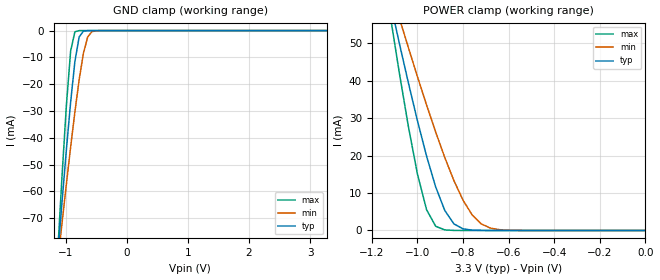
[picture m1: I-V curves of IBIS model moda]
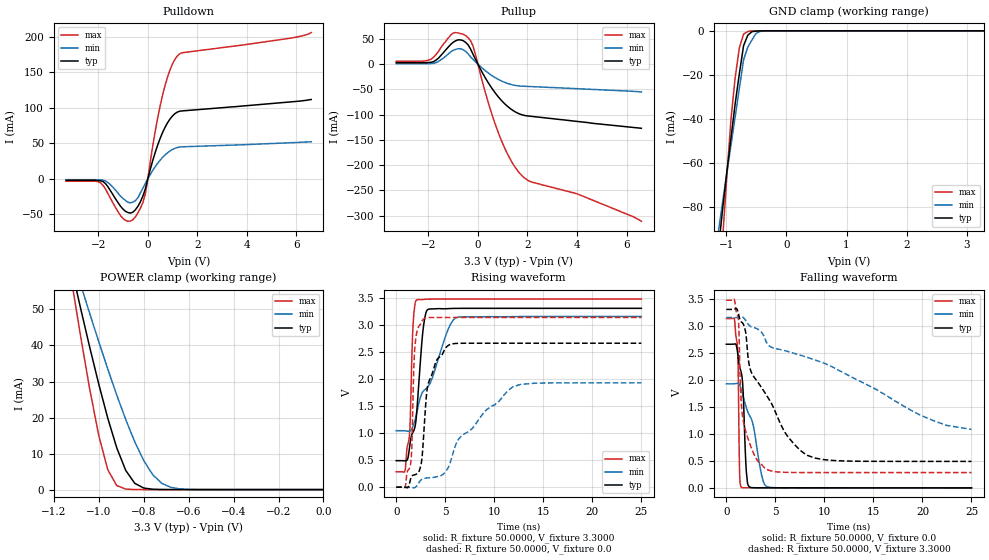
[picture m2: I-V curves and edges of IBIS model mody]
| IBIS (I/O, Buffer, Information, Specification) Model, officially
| electronic behavioral standard for Buffer structures of digital pins.
[IBIS ver]  4.0
[File name] 54ac04_3v3_rev1.ibs
[File Rev]  1.0
[Date]   4 Oct 2017
[Source]   CAD & Design Services (Catania) - STMicroelectronics
[Notes]
  (Note1) This IBIS model is the model of the product with package
   (Flat14 package elements);
  (Note2) This IBIS model is extracted with nominal 3.3V power supply
   (min:3.15V, typ:3.3V, max:3.47V);
  (Note3) This model has few Warnings about the non-monotonicity
   of I-V curves, but they are not indicative of problems
   inside the model;
[Copyright] (c) 2017 STMicroelectronics
|   Component 54AC04
[Component] 54AC04
[Manufacturer] STMicroelectronics
[Package]
| variable   typ   min   max
R_pkg   0.0   0.0   0.0
L_pkg   0.0H   0.0H   0.0H
C_pkg   0.0F   0.0F   0.0F
[Pin]  signal_name   model_name   R_pin   L_pin   C_pin
1   A0   moda   141.0m   4.31nH   1.01pF
2   O0   mody   108.1m   3.05nH   1.04pF
3   A1   moda   90.5m   2.36nH   0.8pF
4   O1   mody   79.7m   1.96nH   0.8pF
5   A2   moda   86.2m   2.16nH   0.8pF
6   O2   mody   101.7m   2.85nH   1.04pF
7   GND   GND   111.0m   3.51nH   1.01pF
8   O5   mody   141.0m   4.31nH   1.01pF
9   A5   moda   112.4m   3.25nH   1.04pF
10   O4   mody   90.5m   2.36nH   0.8pF
11   A4   moda   81.9m   2.06nH   0.8pF
12   O3   mody   84.0m   2.16nH   0.8pF
13   A3   moda   101.7m   2.85nH   1.04pF
14   VCC   POWER   111.0m   3.51nH   1.01pF
| Models and submodels in the file (2): moda (Input), mody (I/O)
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|   Model mod_a
[Model]   moda
Model_type Input
Vinl   =   1.000V
Vinh   =   2.300V
C_comp   0.584pF   0.443pF   0.735pF
[Temperature Range]  25.0000   0.1250k   -55.0000
[Voltage Range]   3.3000V   3.1500V   3.4700V
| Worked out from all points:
|   GND clamp passes 1 mA (typ) near -0.74 V on its own axis
|   POWER clamp passes 1 mA (typ) near -0.82 V on its own axis
[GND_clamp]
|Voltage   I(typ)   I(min)   I(max)
-3.3V     -749mA     -568.4mA   -1.036A
-1.13V    -83.59mA   -86.25mA   -82mA
-1.06V    -63.75mA   -71.67mA   -54.05mA
-990mV    -44.61mA   -57.39mA   -28.12mA
-920mV    -26.72mA   -43.53mA   -7.666mA
-850mV    -11.52mA   -30.35mA   -438.9uA
-780mV    -2.357mA   -18.3mA    -11.16uA
-710mV    -202.6uA   -8.405mA   -269.9nA
-640mV    -13.61uA   -2.367mA   -6.525nA
-570mV    -893.7nA   -396.6uA   -166.8pA
-430mV    -3.851nA   -7.049uA   -9.012pA
3.28V     6.52pA     5.985nA    5.92pA
[POWER_clamp]
|Voltage   I(typ)   I(min)   I(max)
-3.28V    721.1mA    542.9mA    1.005A
-1.12V    61.08mA    64.91mA    57.6mA
-1.08V    50.1mA     56.8mA     42.24mA
-1.04V    39.44mA    48.83mA    27.8mA
-1V       29.27mA    41.04mA    15.03mA
-960mV    19.83mA    33.48mA    5.531mA
-920mV    11.6mA     26.24mA    1.117mA
-880mV    5.324mA    19.45mA    149.5uA
-840mV    1.752mA    13.29mA    18.09uA
-760mV    95.86uA    4.148mA    257.2nA
-680mV    4.309uA    633uA      3.657nA
0V        6.6pA      45.39pA    7.2pA
|   Model mody
[Model]   mody
Model_type I/O
Polarity   Inverting
Vinl   =   1.000V
Vinh   =   2.300V
Vmeas  =   1.650V
Cref   =   50pf
Rref   =   500
C_comp   3.516pF   2.793pF   4.427pF
[Temperature Range]  25.0000   0.1250k   -55.0000
[Voltage Range]   3.3000V   3.1500V   3.4700V
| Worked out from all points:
|   slope of the pulldown table from 0 to 0.495 V, typ, clamps not added: 8.73 ohm
|   slope of the pullup table from 0 to 0.495 V, typ, clamps not added: 11.6 ohm
|   GND clamp passes 1 mA (typ) near -0.60 V on its own axis
|   POWER clamp passes 1 mA (typ) near -0.82 V on its own axis
|   rising waveform, R_fixture 50.0000, V_fixture 3.3000: 20-80 % time 832ps typ, 2.72ns min, 347ps max; typ from 0.489 V to 3.3 V
|   rising waveform, R_fixture 50.0000, V_fixture 0.0: 20-80 % time 1.1ns typ, 4.82ns min, 312ps max; typ from 0 V to 2.66 V
|   falling waveform, R_fixture 50.0000, V_fixture 0.0: 20-80 % time 438ps typ, 1.49ns min, 152ps max; typ from 2.66 V to 0 V
|   falling waveform, R_fixture 50.0000, V_fixture 3.3000: 20-80 % time 3.84ns typ, 14.3ns min, 894ps max; typ from 3.3 V to 0.489 V
[Pulldown]
|Voltage   I(typ)   I(min)   I(max)
-3.3V     -2.144mA   -1.112mA   -3.317mA
-1.9V     -2.784mA   -1.342mA   -5.817mA
-1.6V     -11.54mA   -5.384mA   -21.39mA
-1V       -42.54mA   -27.65mA   -55.74mA
-600mV    -46.82mA   -32.7mA    -57.34mA
-300mV    -32.26mA   -19.88mA   -41.27mA
-100mV    -14.21mA   -6.505mA   -21.18mA
300mV     37.36mA    17.24mA    67.14mA
600mV     65.52mA    30.35mA    118.4mA
900mV     84.46mA    39.35mA    153.8mA
1.2V      94.2mA     44.23mA    173.4mA
6.6V      111.8mA    52.34mA    206mA
[Pullup]
|Voltage   I(typ)   I(min)   I(max)
-3.3V     3.144mA    1.112mA    5.897mA
-2V       3.344mA    1.222mA    7.966mA
-1.6V     11.77mA    5.384mA    24.79mA
-1V       43.44mA    27.55mA    61.74mA
-500mV    43.42mA    25.6mA     56.85mA
-200mV    19.98mA    9.716mA    36.35mA
400mV     -35.28mA   -16.72mA   -72.98mA
900mV     -68.97mA   -31.95mA   -145.1mA
1.7V      -98.8mA    -43.21mA   -216.6mA
2.1V      -102.9mA   -44.16mA   -232mA
4V        -113.2mA   -48.4mA    -256.5mA
6.6V      -126.8mA   -54.96mA   -311mA
[GND_clamp]
|Voltage   I(typ)   I(min)   I(max)
-3.3V     -750.5mA   -569.2mA   -1.049A
-1.13V    -99.8mA    -91.54mA   -122.8mA
-1.06V    -81.6mA    -78.17mA   -95.14mA
-990mV    -64.61mA   -65.1mA    -67.22mA
-920mV    -48.9mA    -52.15mA   -40.51mA
-850mV    -33.2mA    -39.19mA   -21.39mA
-780mV    -19.49mA   -26.19mA   -7.724mA
-710mV    -6.761mA   -13.2mA    -1.514mA
-640mV    -2.019mA   -7.433mA   -302.5uA
-500mV    -143.5uA   -1.107mA   -6.459uA
-360mV    -6.928uA   -54.34uA   -66.17nA
3.28V     2.9pA      17.61pA    1.9pA
[POWER_clamp]
|Voltage   I(typ)   I(min)   I(max)
-3.28V    721.1mA    542.9mA    1.005A
-1.12V    61.08mA    64.91mA    57.6mA
-1.08V    50.1mA     56.8mA     42.24mA
-1.04V    39.44mA    48.83mA    27.8mA
-1V       29.27mA    41.04mA    15.03mA
-960mV    19.83mA    33.48mA    5.531mA
-920mV    11.6mA     26.24mA    1.117mA
-880mV    5.324mA    19.45mA    149.5uA
-840mV    1.752mA    13.29mA    18.09uA
-760mV    95.86uA    4.148mA    257.2nA
-680mV    4.309uA    633uA      3.657nA
0V        6.6pA      45.39pA    7.2pA
[Ramp]
| variable   typ   min   max
dV/dt_r  1.5939/1.1598n   1.1548/4.9334n   1.8787/0.4156n
dV/dt_f  1.6862/3.8631n   1.2323/14.1536n   1.9122/0.9071n
R_load = 50.0000
[Rising Waveform]
R_fixture= 50.0000
V_fixture= 3.3000
V_fixture_min= 3.1500
V_fixture_max= 3.4700
|time   V(typ)   V(min)   V(max)
0s        489.4mV    1.042V     282.9mV
840ps     487.6mV    1.041V     278.3mV
1.32ns    678.4mV    1.033V     907.1mV
1.44ns    841.5mV    1.042V     1.296V
1.72ns    1.016V     1.132V     2.997V
2.08ns    1.356V     1.362V     3.453V
2.72ns    2.874V     1.761V     3.462V
3.24ns    3.281V     1.854V     3.469V
6.08ns    3.299V     3.126V     3.47V
25ns      3.3V       3.15V      3.47V
[Rising Waveform]
R_fixture= 50.0000
V_fixture= 0.0
V_fixture_min= 0.0
V_fixture_max= 0.0
|time   V(typ)   V(min)   V(max)
0s        132.2pV    0V         79.05pV
1.44ns    132.6mV    -3.953mV   396.8mV
1.6ns     206mV      -7.549mV   777.6mV
1.92ns    230.7mV    -5.02mV    2.614V
2.52ns    405.8mV    131.4mV    3.017V
2.84ns    1.073V     162.3mV    3.111V
3.24ns    1.894V     171.3mV    3.13V
5.54ns    2.636V     470.9mV    3.132V
11.86ns   2.657V     1.848V     3.132V
25ns      2.657V     1.924V     3.132V
[Falling Waveform]
R_fixture= 50.0000
V_fixture= 0.0
V_fixture_min= 0.0
V_fixture_max= 0.0
|time   V(typ)   V(min)   V(max)
0s        2.657V     1.924V     3.132V
820ps     2.66V      1.925V     3.13V
1.1ns     2.567V     1.934V     2.684V
1.2ns     2.424V     1.934V     2.27V
1.36ns    2.239V     1.901V     237.4mV
1.54ns    2.119V     1.812V     8.564mV
2.04ns    300.1mV    1.482V     1.983mV
2.42ns    11.62mV    1.322V     2.854mV
4.22ns    1.813mV    17.78mV    1.517mV
25ns      -178.5nV   207.3uV    -429.2nV
[Falling Waveform]
R_fixture= 50.0000
V_fixture= 3.3000
V_fixture_min= 3.1500
V_fixture_max= 3.4700
|time   V(typ)   V(min)   V(max)
0s        3.3V       3.15V      3.47V
1.18ns    3.266V     3.155V     3.172V
1.26ns    3.204V     3.159V     3.023V
1.5ns     3.073V     3.165V     1.644V
1.86ns    2.97V      3.126V     1.128V
2.44ns    2.194V     2.988V     793.7mV
4.06ns    1.724V     2.703V     349.3mV
6.34ns    932.6mV    2.519V     285.6mV
9.06ns    550.1mV    2.365V     283mV
25ns      489.4mV    1.081V     282.9mV
